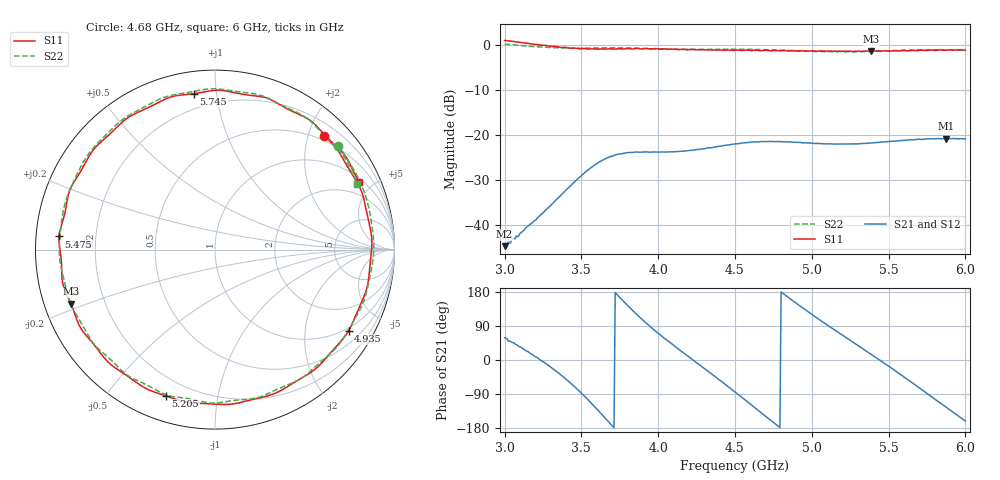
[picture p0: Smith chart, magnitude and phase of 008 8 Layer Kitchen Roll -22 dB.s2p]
!  04/11/2025  15:17:49
! Ref Plane: 0.000 mm
# MHZ S MA R  50
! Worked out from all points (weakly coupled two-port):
!   401 points, 3 GHz to 6 GHz, reference 50 ohm
!   highest |S21| = -20.79 dB at 5.872 GHz (marker M1); lowest = -44.8 dB at 3 GHz (marker M2)
!   lowest |S11| = -1.3 dB at 5.385 GHz (marker M3), VSWR 12.95, Z = 3.99 - j9.04 ohm
!   |S11| at or under -10 dB: nowhere
!   |S22| runs from -1.5 to 0.3 dB; largest |S21 - S12| = 0.0019
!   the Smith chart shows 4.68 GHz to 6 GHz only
!   S11 on the Smith chart (normalised r, x): 4.68 GHz: 0.42, +2.29; 4.935 GHz: 0.89, -3.35; 5.205 GHz: 0.11, -0.71; 5.475 GHz: 0.07, +0.04; 5.745 GHz: 0.12, +0.87; 6 GHz: 1.19, +4.16
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3000  1.136 -113.1  0.005732 59.0  0.005753 60.4  1.034 -116.8
3270  0.9997 179.1  0.01471 -10.1  0.01463 -8.1  0.9544 175.7
3390  0.9532 141.3  0.02338 -46.9  0.02349 -46.6  0.9372 137.5
3502.5  0.9217 98.8  0.03554 -88.6  0.03546 -88.2  0.93 94.9
3607.5  0.9082 54.2  0.04886 -132.3  0.04894 -131.9  0.9341 50.9
3735  0.9166 -2.6  0.0608 171.4  0.061 172.4  0.9408 -4.8
3870  0.9227 -57.3  0.06432 116.3  0.06491 117.3  0.9306 -59.0
4005  0.9102 -104.7  0.06444 69.1  0.06419 69.8  0.912 -105.8
4245  0.8938 -179.3  0.06831 -5.6  0.06849 -4.5  0.8994 179.7
4357.5  0.8869 146.9  0.0727 -39.7  0.07307 -38.6  0.9048 145.0
4500  0.8854 102.5  0.07949 -84.7  0.08008 -83.9  0.9037 99.1
4680  0.8765 46.1  0.08445 -142.5  0.08448 -141.9  0.8976 40.2
4807.5  0.874 6.7  0.08404 177.3  0.08424 178.1  0.8841 -0.7
4935  0.8712 -31.3  0.08189 139.1  0.08191 139.8  0.8691 -39.0
5002.5  0.8688 -50.8  0.08073 119.7  0.08071 120.4  0.8612 -58.3
5205  0.8599 -108.6  0.07905 64.1  0.07927 64.7  0.8466 -113.7
5385  0.8567 -159.4  0.08134 15.6  0.08169 16.4  0.8595 -161.6
5475  0.8724 175.2  0.08375 -9.5  0.08401 -8.8  0.8673 173.7
5505  0.8609 166.7  0.08455 -17.5  0.08504 -16.6  0.8725 165.5
5745  0.877 97.6  0.09026 -86.7  0.09097 -85.8  0.8889 98.1
5872.5  0.8822 61.0  0.09126 -124.2  0.09169 -123.3  0.8872 61.5
6000  0.8854 25.2  0.09042 -161.3  0.09083 -160.7  0.8741 24.9
